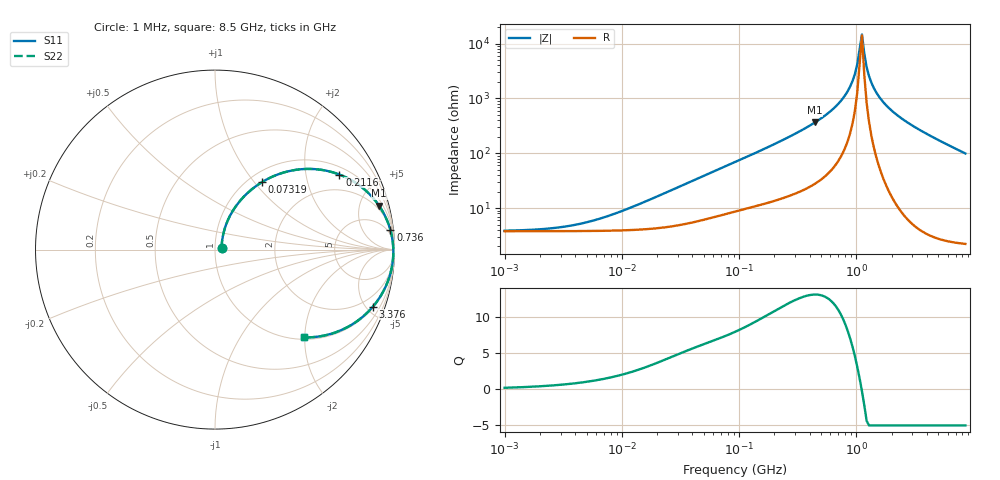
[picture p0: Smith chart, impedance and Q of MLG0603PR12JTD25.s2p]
! S-Parameter Data Generated by TDK Corporation
! Copyright(C) 2025 TDK Corporation.
! All Rights Reserved.
! TDK P/N: MLG0603PR12JTD25 (SMD / SMT Inductor (Coil))
! Property: L=120nH at 300MHz
! Size(LxWxT): 0.6x0.3x0.3mm
! Model Type: s2p (Touchstone File Format Version 1.0)
! Frequency: DC=Yes Start=1MHz Stop=8500MHz 198points Log-sweep
! Model Generated on Feb. 6, 2025
! Terms and conditions regarding TDK Simulation Models:
! 1)This simulation model is being provided solely for informational
!  purposes. Please refer to the specifications of the products in
!  terms of detailed characteristics of such products.
! 2)In no event shall TDK Corporation of any of its subsidiaries be
!  liable for any loss or damage arising, directly or indirectly,
!  from any information contained in this simulation model, including,
!  but not limited to loss or damages arising from any inaccuracies,
!  omissions or errors in connection with such information.
! 3)Any and all copyrights on this simulation model are owned by
!  TDK Corporation.  Duplication or redistribution of this simulation
!  model without prior written permission from TDK Corporation
!  is prohibited.
! 4)This simulation model is subject to any modification or change
!  without any prior notice.
! 5)Neither TDK Corporation nor any of its subsidiaries shall make any
!  warranty, express or implied, including but not limited to the
!  correctness, implied warranties of merchantability and fitness for
!  a particular purpose with respect to this simulation models.
! 6)The use of this simulation model shall be deemed to have consented
!  to the terms and conditions hereof.
! Port Assignments:
!  1 ---@@@--- 2
! Applicable Conditions:
!  Temperature = 25 degC
!  DC Bias Current = 0 A
!  Small Signal Operation
# Hz S MA R 50
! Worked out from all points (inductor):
!   197 points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, 1 MHz to 8.5 GHz, reference 50 ohm
!   read as one part in series: L = 125 nH near 15.95 MHz
!   highest Q = 13.1 at 442.9 MHz (marker M1), where L = 131 nH
!   self-resonance near 1.065 GHz
!   S11 on the Smith chart (normalised r, x): 1 MHz: 1.08, +0.02; 73.19 MHz: 1.15, +1.10; 211.6 MHz: 1.28, +3.11; 736 MHz: 3, +18; 3.376 GHz: 1.08, -5.51; 8.5 GHz: 1.04, -1.98
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1000000  0.03732 11.4  0.9634 -0.4  0.9634 -0.4  0.03732 11.4
4587603  0.05079 41.6  0.9626 -2.0  0.9626 -2.0  0.05079 41.6
2.10461e7  0.1621 66.3  0.9465 -9.0  0.9465 -9.0  0.1621 66.3
4.206225e7  0.298 63.1  0.9051 -17.1  0.9051 -17.1  0.298 63.1
7.319294e7  0.4592 55.1  0.8279 -27.1  0.8279 -27.1  0.4592 55.1
9.219544e7  0.5373 50.6  0.7789 -32.2  0.7789 -32.2  0.5373 50.6
2.116287e8  0.8095 31.1  0.5187 -53.7  0.5187 -53.7  0.8095 31.1
4.229561e8  0.941 15.9  0.2742 -69.8  0.2742 -69.8  0.941 15.9
4.429384e8  0.9463 15.0  0.2593 -70.7  0.2593 -70.7  0.9463 15.0
7.359901e8  0.9836 6.2  0.1093 -78.2  0.1093 -78.2  0.9836 6.2
8.852465e8  0.9898 3.4  0.05971 -78.5  0.05971 -78.5  0.9898 3.4
9.708683e8  0.9918 2.0  0.03554 -75.7  0.03554 -75.7  0.9918 2.0
1.016736e9  0.9925 1.3  0.02369 -71.0  0.02369 -71.0  0.9925 1.3
1.115076e9  0.9935 -0.1  0.006764 14.5  0.006764 14.5  0.9935 -0.1
1.167757e9  0.9937 -0.8  0.01522 65.0  0.01522 65.0  0.9937 -0.8
1.222927e9  0.9937 -1.5  0.02676 75.6  0.02676 75.6  0.9937 -1.5
1.34121e9  0.9932 -2.9  0.051 80.9  0.051 80.9  0.9932 -2.9
1.540426e9  0.9911 -5.1  0.08857 81.7  0.08857 81.7  0.9911 -5.1
1.940355e9  0.9836 -8.9  0.1547 79.5  0.1547 79.5  0.9836 -8.9
3.37643e9  0.9354 -19.9  0.3397 69.3  0.3397 69.3  0.9354 -19.9
5.610304e9  0.8319 -32.8  0.5411 56.3  0.5411 56.3  0.8319 -32.8
8.5e9  0.6964 -44.6  0.7022 44.1  0.7022 44.1  0.6964 -44.6
